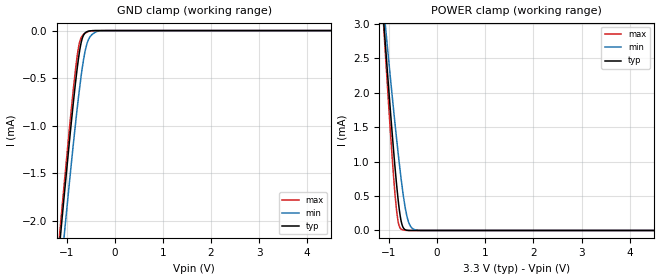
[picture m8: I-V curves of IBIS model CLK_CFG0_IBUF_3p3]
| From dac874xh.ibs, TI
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|   CLK_CFG0_IBUF_3p3 Model
[Model]   CLK_CFG0_IBUF_3p3
Model_type   Input
Vinl = 0.99
Vinh = 2.31
|   typ   min   max
C_comp   1.45519E-13  3.62136E-14  2.16738E-13
| Where nom  PVT is Nominal Process, 3.3V, 27C
|   Fast PVT is Strong Process,  3.6V, -40C
|   Slow PVT is Weak Process,   3.0V, 150C
[Model spec]
|subparameter
Vinl   0.99   0.9   1.08
Vinh   2.31   2.1   2.52
[Voltage Range]   3.3   3   3.6
[Temperature Range]   27   150   -40
[Power Clamp Reference]   3.3   3   3.6
[GND Clamp Reference]   0   0   0
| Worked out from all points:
|   GND clamp passes 1 mA (typ) near -0.91 V on its own axis
|   POWER clamp passes 1 mA (typ) near -0.89 V on its own axis
[GND Clamp]
|   Voltage   I(typ)   I(min)   I(max)
-3.3V     -14.66mA   -14.73mA   -14.82mA
-1.251V   -2.851mA   -3.236mA   -2.747mA
-1.102V   -2.031mA   -2.441mA   -1.912mA
-1.053V   -1.763mA   -2.181mA   -1.639mA
-904.2mV  -984.9uA   -1.42mA    -845.2uA
-775.5mV  -386.5uA   -807.4uA   -256.6uA
-726mV    -207.6uA   -594.9uA   -117.3uA
-676.5mV  -87.91uA   -405.4uA   -57.67uA
-567.6mV  -10.34uA   -126uA     -13.55uA
-399.3mV  -90.59nA   -16.34uA   -99.85nA
-181.5mV  0A         -35.72nA   0A
6.6V      0A         0A         0A
[POWER Clamp]
|   Voltage   I(typ)   I(min)   I(max)
-3.3V     25.21mA    20.41mA    29.38mA
-1.112V   3.041mA    3.239mA    2.971mA
-1.092V   2.853mA    3.092mA    2.748mA
-1.023V   2.204mA    2.586mA    1.98mA
-933.9mV  1.402mA    1.95mA     1.052mA
-874.5mV  906.6uA    1.542mA    515.1uA
-805.2mV  410.3uA    1.089mA    107.9uA
-726mV    76.02uA    624.7uA    10.52uA
-656.7mV  8.351uA    304uA      1.833uA
-587.4mV  749.8nA    109.2uA    225nA
-399.3mV  0A         2.282uA    0A
6.6V      0A         0A         0A
